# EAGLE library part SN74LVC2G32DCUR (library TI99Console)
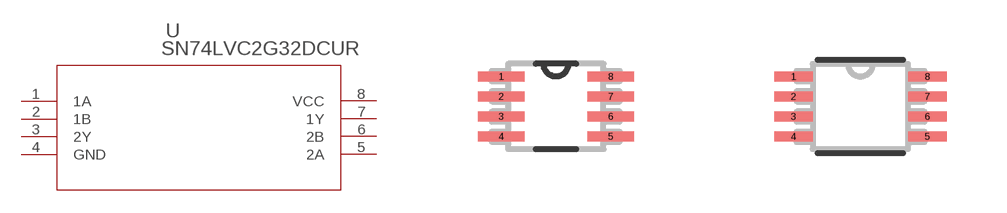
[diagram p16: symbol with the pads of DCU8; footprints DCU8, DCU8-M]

Designator prefix U

## SN74LVC2G32DCUR (COPYRIGHT: Copyright (C) 2022 Ultra Librarian. All rights reserved.; DIGI-KEY_PART_NUMBER_1: 296-13268-1-ND; DIGI-KEY_PART_NUMBER_2: 296-13268-2-ND; DIGI-KEY_PART_NUMBER_3: 296-13268-6-ND; DIGI-KEY_PART_NUMBER_4: 2156-SN74LVC2G32DCUR-ND; MANUFACTURER_PART_NUMBER: SN74LVC2G32DCUR; MFR_NAME: Texas Instruments)  [DCU8]
1  1A  in
2  1B  in
3  2Y  out
4  GND  pwr
5  2A  in
6  2B  in
7  1Y  out
8  VCC  pwr

## SN74LVC2G32DCURDCU8-M (COPYRIGHT: Copyright (C) 2022 Ultra Librarian. All rights reserved.; DIGI-KEY_PART_NUMBER_1: 296-13268-1-ND; DIGI-KEY_PART_NUMBER_2: 296-13268-2-ND; DIGI-KEY_PART_NUMBER_3: 296-13268-6-ND; DIGI-KEY_PART_NUMBER_4: 2156-SN74LVC2G32DCUR-ND; MANUFACTURER_PART_NUMBER: SN74LVC2G32DCUR; MFR_NAME: Texas Instruments)  [DCU8-M]
Pads as for DCU8

## SN74LVC2G32DCURDCU8-L (COPYRIGHT: Copyright (C) 2022 Ultra Librarian. All rights reserved.; DIGI-KEY_PART_NUMBER_1: 296-13268-1-ND; DIGI-KEY_PART_NUMBER_2: 296-13268-2-ND; DIGI-KEY_PART_NUMBER_3: 296-13268-6-ND; DIGI-KEY_PART_NUMBER_4: 2156-SN74LVC2G32DCUR-ND; MANUFACTURER_PART_NUMBER: SN74LVC2G32DCUR; MFR_NAME: Texas Instruments)  [DCU8-L]
Pads as for DCU8

## Footprint DCU8 (pad centres in mm)
smd 1.168 x 0.254: 1 -1.372,0.75; 2 -1.372,0.25; 3 -1.372,-0.25; 4 -1.372,-0.75; 5 1.372,-0.75; 6 1.372,-0.25; 7 1.372,0.25; 8 1.372,0.75

## Footprint DCU8-M (pad centres in mm)
smd 0.965 x 0.254: 1 -1.676,0.75; 2 -1.676,0.25; 3 -1.676,-0.25; 4 -1.676,-0.75; 5 1.676,-0.75; 6 1.676,-0.25; 7 1.676,0.25; 8 1.676,0.75

## Footprint DCU8-L (pad centres in mm)
smd 0.559 x 0.203: 1 -1.473,0.75; 2 -1.473,0.25; 3 -1.473,-0.25; 4 -1.473,-0.75; 5 1.473,-0.75; 6 1.473,-0.25; 7 1.473,0.25; 8 1.473,0.75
